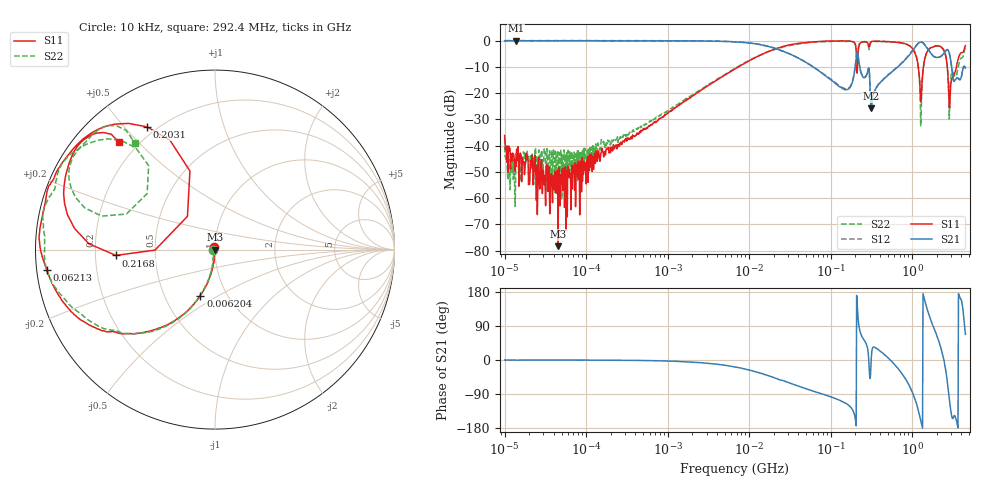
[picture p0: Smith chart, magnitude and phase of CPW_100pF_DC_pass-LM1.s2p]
!Siglent Technologies,SNA5004A,SNA5XCED5R0097,V1.0.0.2.10.R9
!Date: 2024-10-29 17:16:16
!Data & Calibration Information:
!Freq	S11:F2(ON)	S21:F2(ON)	S12:F2(ON)	S22:F2(ON)
# Hz S DB R 50
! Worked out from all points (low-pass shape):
!   1001 points, 10 kHz to 4.5 GHz, reference 50 ohm
!   highest |S21| = 0.00 dB at 13.85 kHz (marker M1); lowest = -25.7 dB at 312.1 MHz (marker M2)
!   |S21| within 3 dB of the highest: start of sweep to 21.07 MHz; 1.062 GHz to 1.538 GHz (475.7 MHz wide, 36.6 % of centre)
!   lowest |S11| = -78.3 dB at 45.27 kHz (marker M3), VSWR 1.00, Z = 50 + j0.00995 ohm
!   |S11| at or under -10 dB: start of sweep to 7.386 MHz; 1.189 GHz to 1.374 GHz (185.7 MHz wide, 14.5 % of centre); 2.695 GHz to 3.494 GHz (799.8 MHz wide, 25.8 % of centre)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
!   |S22| runs from -63.2 to -0.2 dB; largest |S21 - S12| = 0.023
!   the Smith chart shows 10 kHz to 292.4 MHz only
!   S11 on the Smith chart (normalised r, x): 10 kHz: 0.99, +0.03; 6.204 MHz: 0.75, -0.42; 62.13 MHz: 0.03, -0.06; 203.1 MHz: 0.16, +0.58; 216.8 MHz: 0.29, -0.03; 292.4 MHz: 0.13, +0.44
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10000  -36.12 117.1  -0.15 0.1  -0.04 0.2  -37.37 -161.4
13846.19  -47.89 -33.2  0.00 -0.2  0.06 -0.3  -43.10 -48.3
45266.06  -78.30 54.9  -0.06 -0.0  -0.00 0.0  -46.53 164.6
87919.76  -57.52 -119.9  -0.06 -0.2  -0.00 -0.2  -44.24 -139.5
772988.4  -29.94 -96.8  -0.08 -2.1  -0.02 -2.1  -28.77 -100.2
6204217  -11.42 -107.5  -0.41 -16.9  -0.37 -16.9  -11.19 -108.3
6708204  -10.77 -108.9  -0.47 -18.2  -0.42 -18.2  -10.59 -109.3
5.897837e7  -0.55 -171.5  -9.75 -81.1  -9.64 -81.0  -0.56 -171.4
6.213061e7  -0.50 -173.1  -10.20 -82.7  -10.09 -82.6  -0.50 -172.9
1.56561e8  -0.14 154.5  -18.68 -115.2  -18.30 -114.8  -0.28 155.6
2.031178e8  -2.14 118.9  -8.32 -162.2  -8.11 -161.9  -1.89 130.8
2.167774e8  -5.15 -176.6  -5.61 111.5  -5.43 111.7  -3.63 163.6
2.924407e8  -1.87 131.8  -10.44 5.0  -10.36 5.2  -2.55 126.9
3.121073e8  -0.52 138.3  -25.73 -17.6  -25.64 -17.3  -0.68 140.0
5.185364e8  -0.42 95.1  -12.85 3.4  -12.76 3.7  -0.37 93.6
9.314806e8  -1.98 23.5  -5.34 -69.4  -5.06 -68.9  -1.98 20.7
1.323764e9  -15.62 74.2  -0.69 -174.6  -0.61 -174.0  -16.24 93.6
1.856924e9  -2.30 -8.7  -6.17 83.6  -6.10 84.3  -2.24 -7.6
2.440684e9  -3.65 -96.0  -4.89 1.9  -4.82 2.8  -3.56 -91.9
2.928576e9  -20.64 -94.7  -6.30 -121.9  -6.29 -120.8  -17.38 -59.1
3.560038e9  -8.63 68.2  -14.28 -168.0  -14.23 -166.3  -12.08 105.3
4.5e9  -1.94 -36.6  -10.44 67.8  -10.54 64.7  -2.41 -23.9
